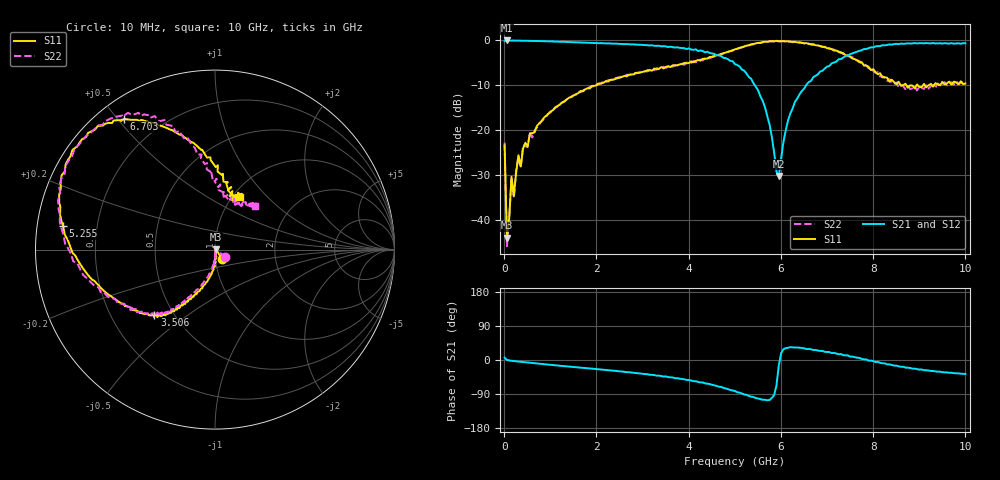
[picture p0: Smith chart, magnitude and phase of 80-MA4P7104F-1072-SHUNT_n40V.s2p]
!Agilent Technologies,E8364C,MY48140145,A.09.42.15
!Agilent E8364C: A.09.42.15
!Date: Wednesday, December 02, 2020 11:12:10
!Correction: S11(Full 2 Port(1,2))
!S21(Full 2 Port(1,2))
!S12(Full 2 Port(1,2))
!S22(Full 2 Port(1,2))
!S2P File: Measurements: S11, S21, S12, S22:
# Hz S  dB  R 50
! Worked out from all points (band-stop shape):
!   201 points, 10 MHz to 10 GHz, reference 50 ohm
!   highest |S21| = -0.19 dB at 59.95 MHz (marker M1); lowest = -30.2 dB at 5.954 GHz (marker M2)
!   |S21| within 3 dB of the highest: start of sweep to 4.559 GHz; 7.51 GHz to end of sweep
!   lowest |S11| = -43.9 dB at 59.95 MHz (marker M3), VSWR 1.01, Z = 50.6 + j0.0686 ohm
!   |S11| at or under -10 dB: start of sweep to 2.022 GHz; 8.589 GHz to 8.668 GHz (78.71 MHz wide, 0.912 % of centre); 8.713 GHz to 8.948 GHz (234.6 MHz wide, 2.66 % of centre)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
!   |S22| runs from -45.8 to -0.3 dB; largest |S21 - S12| = 0.031
!   S11 on the Smith chart (normalised r, x): 10 MHz: 1.08, -0.12; 3.506 GHz: 0.39, -0.38; 5.255 GHz: 0.08, +0.08; 6.703 GHz: 0.08, +0.52; 10 GHz: 1.08, +0.71
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1e7  -23.47 -53.3  -0.33 6.2  -0.33 4.4  -22.87 -35.9
5.995e7  -43.92 6.1  -0.19 0.2  -0.20 -0.0  -45.79 -3.8
1.099e8  -39.53 -83.1  -0.22 -1.2  -0.21 -1.3  -39.50 -82.1
1.5985e8  -30.38 -85.0  -0.21 -2.0  -0.21 -2.1  -30.50 -82.5
2.098e8  -34.70 -73.8  -0.21 -2.7  -0.21 -2.8  -35.16 -86.6
3.097e8  -25.63 -87.5  -0.24 -4.1  -0.24 -4.2  -26.14 -86.4
3.5965e8  -28.14 -78.6  -0.24 -4.9  -0.23 -4.8  -28.43 -91.7
4.096e8  -24.16 -90.9  -0.24 -5.4  -0.26 -5.4  -23.45 -90.6
8.5915e8  -17.34 -97.9  -0.36 -11.0  -0.34 -10.9  -17.58 -100.8
1.7083e9  -11.47 -113.3  -0.64 -20.8  -0.63 -20.6  -11.31 -117.0
3.35665e9  -6.46 -130.3  -1.35 -41.2  -1.39 -42.1  -6.45 -130.6
3.5065e9  -6.06 -132.6  -1.50 -43.3  -1.47 -44.7  -6.25 -132.7
4.4056e9  -4.20 -152.8  -2.68 -62.3  -2.67 -63.5  -4.19 -151.4
5.005e9  -2.16 -177.7  -5.46 -82.0  -5.36 -81.8  -2.26 -174.3
5.25475e9  -1.35 171.3  -7.54 -91.8  -7.45 -92.3  -1.43 174.4
5.65435e9  -0.45 154.2  -14.97 -104.9  -14.90 -104.9  -0.51 155.3
5.95405e9  -0.36 143.2  -30.25 -15.2  -30.28 -15.2  -0.38 142.0
6.2038e9  -0.45 135.6  -16.39 33.9  -16.39 34.0  -0.45 133.2
6.7033e9  -1.04 124.8  -8.33 26.2  -8.29 27.8  -1.13 121.1
7.5025e9  -3.74 105.3  -3.22 8.9  -3.16 10.9  -3.92 105.3
8.35165e9  -9.31 77.7  -1.06 -11.7  -1.16 -12.3  -8.76 85.3
1e10  -9.73 64.6  -0.83 -36.8  -0.82 -36.9  -9.62 47.5
